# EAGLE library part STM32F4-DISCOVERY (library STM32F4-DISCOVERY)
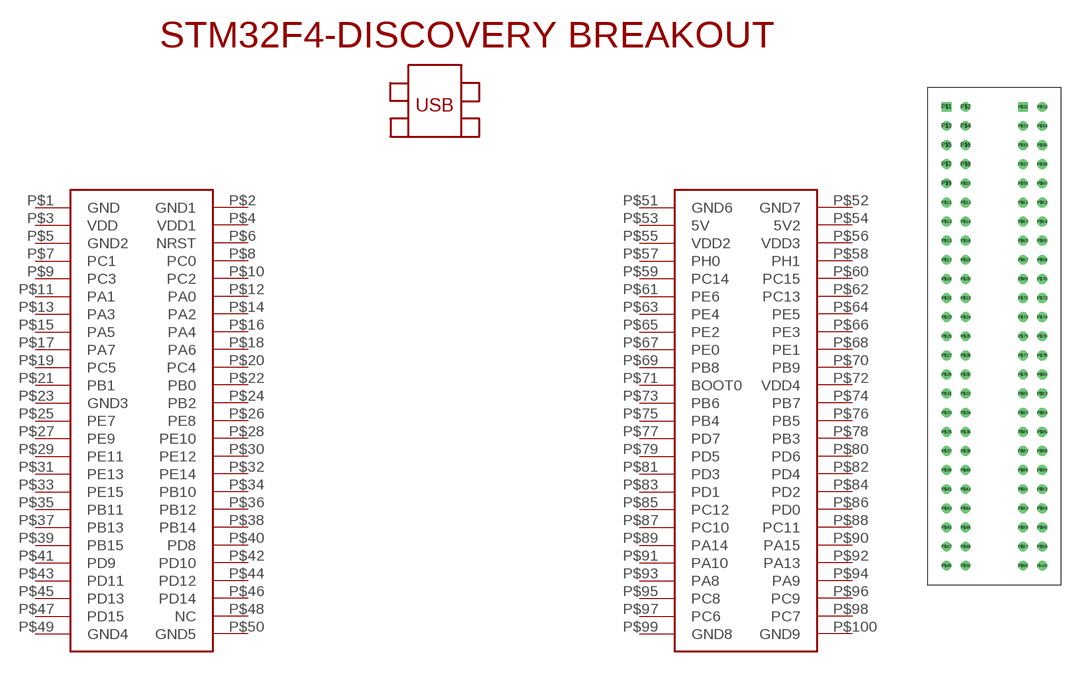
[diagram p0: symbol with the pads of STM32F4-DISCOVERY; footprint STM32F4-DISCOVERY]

Designator prefix -

## STM32F4-DISCOVERY  [STM32F4-DISCOVERY]
P$1  GND
P$2  GND1
P$3  VDD
P$4  VDD1
P$5  GND2
P$6  NRST
P$7  PC1
P$8  PC0
P$9  PC3
P$10  PC2
P$11  PA1
P$12  PA0
P$13  PA3
P$14  PA2
P$15  PA5
P$16  PA4
P$17  PA7
P$18  PA6
P$19  PC5
P$20  PC4
P$21  PB1
P$22  PB0
P$23  GND3
P$24  PB2
P$25  PE7
P$26  PE8
P$27  PE9
P$28  PE10
P$29  PE11
P$30  PE12
P$31  PE13
P$32  PE14
P$33  PE15
P$34  PB10
P$35  PB11
P$36  PB12
P$37  PB13
P$38  PB14
P$39  PB15
P$40  PD8
P$41  PD9
P$42  PD10
P$43  PD11
P$44  PD12
P$45  PD13
P$46  PD14
P$47  PD15
P$48  NC
P$49  GND4
P$50  GND5
P$51  GND6
P$52  GND7
P$53  5V
P$54  5V2
P$55  VDD2
P$56  VDD3
P$57  PH0
P$58  PH1
P$59  PC14
P$60  PC15
P$61  PE6
P$62  PC13
P$63  PE4
P$64  PE5
P$65  PE2
P$66  PE3
P$67  PE0
P$68  PE1
P$69  PB8
P$70  PB9
P$71  BOOT0
P$72  VDD4
P$73  PB6
P$74  PB7
P$75  PB4
P$76  PB5
P$77  PD7
P$78  PB3
P$79  PD5
P$80  PD6
P$81  PD3
P$82  PD4
P$83  PD1
P$84  PD2
P$85  PC12
P$86  PD0
P$87  PC10
P$88  PC11
P$89  PA14
P$90  PA15
P$91  PA10
P$92  PA13
P$93  PA8
P$94  PA9
P$95  PC8
P$96  PC9
P$97  PC6
P$98  PC7
P$99  GND8
P$100  GND9

## Footprint STM32F4-DISCOVERY (pad centres in mm)
drill 0.8 square: P$1 -27.94,30.48; P$51 -17.78,30.48
drill 0.8: P$2 -25.4,30.48; P$3 -27.94,27.94; P$4 -25.4,27.94; P$5 -27.94,25.4; P$6 -25.4,25.4; P$7 -27.94,22.86; P$8 -25.4,22.86; P$9 -27.94,20.32; P$10 -25.4,20.32; P$11 -27.94,17.78; P$12 -25.4,17.78; P$13 -27.94,15.24; P$14 -25.4,15.24; P$15 -27.94,12.7; P$16 -25.4,12.7; P$17 -27.94,10.16; P$18 -25.4,10.16; P$19 -27.94,7.62; P$20 -25.4,7.62; P$21 -27.94,5.08; P$22 -25.4,5.08; P$23 -27.94,2.54; P$24 -25.4,2.54; P$25 -27.94,0; P$26 -25.4,0; P$27 -27.94,-2.54; P$28 -25.4,-2.54; P$29 -27.94,-5.08; P$30 -25.4,-5.08; P$31 -27.94,-7.62; P$32 -25.4,-7.62; P$33 -27.94,-10.16; P$34 -25.4,-10.16; P$35 -27.94,-12.7; P$36 -25.4,-12.7; P$37 -27.94,-15.24; P$38 -25.4,-15.24; P$39 -27.94,-17.78; P$40 -25.4,-17.78; P$41 -27.94,-20.32; P$42 -25.4,-20.32; P$43 -27.94,-22.86; P$44 -25.4,-22.86; P$45 -27.94,-25.4; P$46 -25.4,-25.4; P$47 -27.94,-27.94; P$48 -25.4,-27.94; P$49 -27.94,-30.48; P$50 -25.4,-30.48; P$52 -15.24,30.48; P$53 -17.78,27.94; P$54 -15.24,27.94; P$55 -17.78,25.4; P$56 -15.24,25.4; P$57 -17.78,22.86; P$58 -15.24,22.86; P$59 -17.78,20.32; P$60 -15.24,20.32; P$61 -17.78,17.78; P$62 -15.24,17.78; P$63 -17.78,15.24; P$64 -15.24,15.24; P$65 -17.78,12.7; P$66 -15.24,12.7; P$67 -17.78,10.16; P$68 -15.24,10.16; P$69 -17.78,7.62; P$70 -15.24,7.62; P$71 -17.78,5.08; P$72 -15.24,5.08; P$73 -17.78,2.54; P$74 -15.24,2.54; P$75 -17.78,0; P$76 -15.24,0; P$77 -17.78,-2.54; P$78 -15.24,-2.54; P$79 -17.78,-5.08; P$80 -15.24,-5.08; P$81 -17.78,-7.62; P$82 -15.24,-7.62; P$83 -17.78,-10.16; P$84 -15.24,-10.16; P$85 -17.78,-12.7; P$86 -15.24,-12.7; P$87 -17.78,-15.24; P$88 -15.24,-15.24; P$89 -17.78,-17.78; P$90 -15.24,-17.78; P$91 -17.78,-20.32; P$92 -15.24,-20.32; P$93 -17.78,-22.86; P$94 -15.24,-22.86; P$95 -17.78,-25.4; P$96 -15.24,-25.4; P$97 -17.78,-27.94; P$98 -15.24,-27.94; P$99 -17.78,-30.48; P$100 -15.24,-30.48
